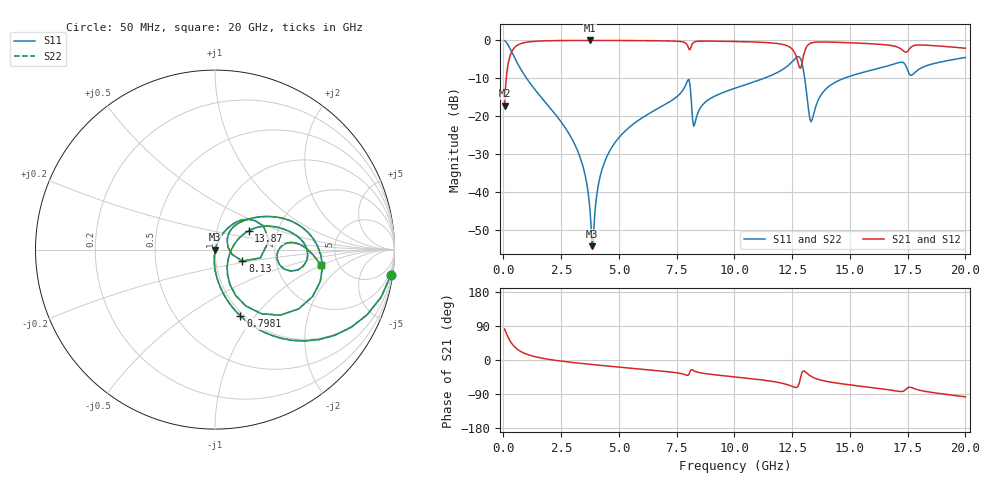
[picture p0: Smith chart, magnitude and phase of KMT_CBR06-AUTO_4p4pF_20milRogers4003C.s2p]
! Data measured by Modelithics Inc. support@modelithics.com 813-866-6335
! KEMET CBR06-AUTO 4.4pF, Pad Width= 0.851mm, Pad Length= 0.64mm, Pad Gap= 0.62mm, 20mil Rogers 4003C substrate Data, January 2022
# hz S ma R 50
! 2 Port Network Data from SP1.SP block
! freq  magS11  angS11  magS21  angS21  magS12  angS12  magS22  angS22
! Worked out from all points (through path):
!   401 points, 50 MHz to 20 GHz, reference 50 ohm
!   highest |S21| = -0.02 dB at 3.741 GHz (marker M1); lowest = -17.2 dB at 50 MHz (marker M2)
!   group delay of S21, straight-line fit = 15.4 ps
!   lowest |S11| = -54.1 dB at 3.841 GHz (marker M3), VSWR 1.00, Z = 50.2 - j0.117 ohm
!   |S11| at or under -10 dB: 1.006 GHz to 11.27 GHz (10.26 GHz wide, 167 % of centre); 13.04 GHz to 14.74 GHz (1.693 GHz wide, 12.2 % of centre)
!   |S22| runs from -54.1 to -0.1 dB; largest |S21 - S12| = 0
!   S11 on the Smith chart (normalised r, x): 50 MHz: 1, -14; 798.1 MHz: 0.97, -0.85; 8.13 GHz: 1.35, -0.18; 13.87 GHz: 1.42, +0.31; 20 GHz: 3.66, -1.00
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5e7  0.9904 -8.1  0.138 81.9  0.138 81.9  0.9904 -8.1
2.99375e8  0.7657 -40.9  0.6423 49.0  0.6423 49.0  0.7657 -40.9
7.98125e8  0.3956 -69.1  0.9174 20.8  0.9174 20.8  0.3956 -69.1
3.391625e9  0.02481 -95.3  0.9979 -9.2  0.9979 -9.2  0.02481 -95.3
3.74075e9  0.00617 -84.7  0.9981 -11.4  0.9981 -11.4  0.00617 -84.7
3.8405e9  0.001965 -36.6  0.9981 -12.0  0.9981 -12.0  0.001965 -36.6
4.189625e9  0.01634 69.4  0.9979 -14.0  0.9979 -14.0  0.01634 69.4
4.6385e9  0.03686 70.3  0.9972 -16.6  0.9972 -16.6  0.03686 70.3
6.73325e9  0.1295 60.2  0.9883 -28.4  0.9883 -28.4  0.1295 60.2
7.980125e9  0.2995 25.9  0.8423 -40.8  0.8423 -40.8  0.2995 25.9
8.12975e9  0.166 -22.8  0.8339 -25.7  0.8339 -25.7  0.166 -22.8
8.279375e9  0.07893 30.1  0.9576 -29.6  0.9576 -29.6  0.07893 30.1
8.778125e9  0.1576 51.1  0.9799 -36.3  0.9799 -36.3  0.1576 51.1
1.0025e10  0.2352 44.2  0.9669 -44.6  0.9669 -44.6  0.2352 44.2
1.22195e10  0.4413 21.9  0.8641 -63.8  0.8641 -63.8  0.4413 21.9
1.276812e10  0.6129 -16.9  0.492 -67.6  0.492 -67.6  0.6129 -16.9
1.296762e10  0.4398 -54.2  0.5837 -29.1  0.5837 -29.1  0.4398 -54.2
1.336662e10  0.09072 -0.7  0.9322 -44.7  0.9322 -44.7  0.09072 -0.7
1.386538e10  0.2139 29.1  0.9542 -54.9  0.9542 -54.9  0.2139 29.1
1.670825e10  0.4685 8.7  0.8631 -78.9  0.8631 -78.9  0.4685 8.7
1.765588e10  0.3472 -4.1  0.8186 -72.6  0.8186 -72.6  0.3472 -4.1
2e10  0.5961 -8.5  0.7883 -97.2  0.7883 -97.2  0.5961 -8.5
